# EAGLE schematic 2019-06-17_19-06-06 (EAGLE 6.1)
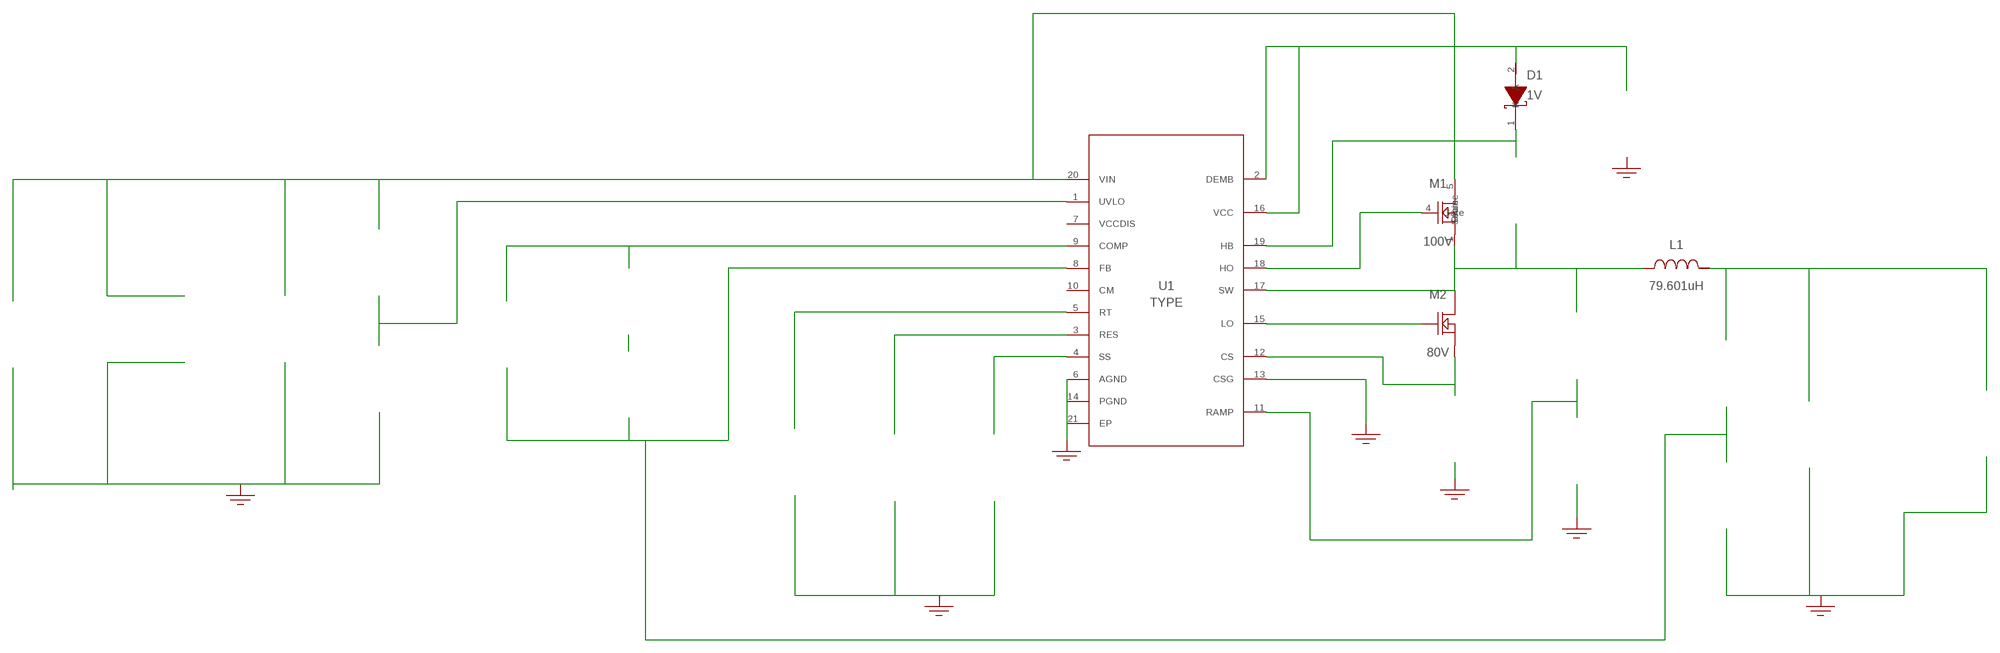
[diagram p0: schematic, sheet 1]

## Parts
CBOOT  100nF  GRM155R71A104KA01DGRM155R71A104KA01D  [0402]  (not placed on a sheet)
CCOMP1  820pF  CL05C821JB5NNNCCL05C821JB5NNNC  [0402]  (not placed on a sheet)
CCOMP2  680pF  GRM033R71C681KA01DGRM033R71C681KA01D  [0201]  (not placed on a sheet)
CIN  15uF  100SXV15M100SXV15M  [CAPSMT_62_E12]  (not placed on a sheet)
CIN_2  15uF  100SXV15M100SXV15M  [CAPSMT_62_E12]  (not placed on a sheet)
CINX  100nF  C2012X7R2A104K125AAC2012X7R2A104K125AA  [0805]  (not placed on a sheet)
COUT  22uF  EEE-FK1J220XPEEE-FK1J220XP  [SM_RADIAL_D8]  (not placed on a sheet)
CRAMP  820pF  GRM033R71E821KA01DGRM033R71E821KA01D  [0201]  (not placed on a sheet)
CRES  470nF  TMK212BJ474KD-TTMK212BJ474KD-T  [0805]  (not placed on a sheet)
CSS  15nF  CGA4F2C0G1H153J085AACGA4F2C0G1H153J085AA  [0805]  (not placed on a sheet)
CVCC  470nF  TMK212BJ474KD-TTMK212BJ474KD-T  [0805]  (not placed on a sheet)
D1  1V  CDBW46-GCDBW46-G  [SOD-123]
GND1  WB_GND  WB_GNDWB_GND  [WB_GND]
GND2  WB_GND  WB_GNDWB_GND  [WB_GND]
GND3  WB_GND  WB_GNDWB_GND  [WB_GND]
GND4  WB_GND  WB_GNDWB_GND  [WB_GND]
GND5  WB_GND  WB_GNDWB_GND  [WB_GND]
GND6  WB_GND  WB_GNDWB_GND  [WB_GND]
GND7  WB_GND  WB_GNDWB_GND  [WB_GND]
GND8  WB_GND  WB_GNDWB_GND  [WB_GND]
IOUT  WB_CURRENT_LOAD  WB_CURRENT_LOADWB_CURRENT_LOAD  [WB_CURRENT_LOAD]  (not placed on a sheet)
L1  79.601uH  CUSTOM1CUSTOM1  [GEN_Ind]
M1  100V  CSD19537Q3CSD19537Q3  [DQG0008A]
M2  80V  BSC117N08NS5ATMA1BSC117N08NS5ATMA1  [PG-TDSON-8]
RCOMP  40.2k  CRCW040240K2FKEDCRCW040240K2FKED  [0402]  (not placed on a sheet)
RFB1  910  RC0603FR-07910RLRC0603FR-07910RL  [0603]  (not placed on a sheet)
RFB2  47k  RC0603FR-0747KLRC0603FR-0747KL  [0603]  (not placed on a sheet)
RRAMP  806k  CRCW0603806KFKEACRCW0603806KFKEA  [0603]  (not placed on a sheet)
RSENSE  12m  CSR1206FK12L0CSR1206FK12L0  [1206]  (not placed on a sheet)
RT  9.31k  CRCW04029K31FKEDCRCW04029K31FKED  [0402]  (not placed on a sheet)
RUV1  1.3k  CRCW04021K30FKEDCRCW04021K30FKED  [0402]  (not placed on a sheet)
RUV2  54.9k  CRCW060354K9FKEACRCW060354K9FKEA  [0603]  (not placed on a sheet)
U1  LM5117PMHX/NOPB  LM5117PMHX/NOPBLM5117PMHX/NOPB  [PWP0020A]
VIN  WB_BATTERY  WB_BATTERYWB_BATTERY  [WB_BATTERY]  (not placed on a sheet)

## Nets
0: Cin.-@2 Cin_2.-@2 Cinx.2@2 Cout.-@2 Cramp.2@2 Cres.2@2 Css.2@2 Cvcc.2@2 GND1.1 GND2.1 GND3.1 GND4.1 GND5.1 GND6.1 GND7.1 GND8.1 Iout.-@2 Rfb1.2@2 Rsense.2@2 Rt.2@2 Ruv1.2@2 U1.6(AGND) U1.13(CSG) U1.14(PGND) U1.21(EP) Vin.-@2
1: Cvcc.1@1 D1.2(A) U1.2(DEMB) U1.16(VCC)
2: Ccomp2.2@2 Rcomp.2@2 Rfb1.1@1 Rfb2.2@2 U1.8(FB)
3: Cboot.2@2 L1.1 M1.1(Source) M1.2(Source) M1.3(Source) M2.5(Drain) M2.6(Drain) M2.7(Drain) M2.8(Drain) M2.9(Drain) Rramp.1@1 U1.17(SW)
4: Cboot.1@1 D1.1(K) U1.19(HB)
5: Cin.+@1 Cin_2.+@1 Cinx.1@1 M1.5(Drain) M1.6(Drain) M1.7(Drain) M1.8(Drain) M1.9(Drain) Ruv2.1@1 U1.20(VIN) Vin.+@1
6: Cramp.1@1 Rramp.2@2 U1.11(RAMP)
7: M2.1(Source) M2.2(Source) M2.3(Source) Rsense.1@1 U1.12(CS)
8: Cout.+@1 Iout.+@1 L1.2 Rfb2.1@1
9: Rt.1@1 U1.5(RT)
10: Ruv1.1@1 Ruv2.2@2 U1.1(UVLO)
11: Ccomp1.1@1 Ccomp2.1@1 U1.9(COMP)
12: Cres.1@1 U1.3(RES)
13: Css.1@1 U1.4(SS)
14: M1.4(Gate) U1.18(HO)
15: Ccomp1.2@2 Rcomp.1@1
16: M2.4(Gate) U1.15(LO)
Unconnected: CBOOT.1 CBOOT.2 CCOMP1.1 CCOMP1.2 CCOMP2.1 CCOMP2.2 CIN.1(+) CIN.2(-) CIN_2.1(+) CIN_2.2(-) CINX.1 CINX.2 COUT.1(+) COUT.2(-) CRAMP.1 CRAMP.2 CRES.1 CRES.2 CSS.1 CSS.2 CVCC.1 CVCC.2 IOUT.1(+) IOUT.2(-) RCOMP.1 RCOMP.2 RFB1.1 RFB1.2 RFB2.1 RFB2.2 RRAMP.1 RRAMP.2 RSENSE.1 RSENSE.2 RT.1 RT.2 RUV1.1 RUV1.2 RUV2.1 RUV2.2 U1.7(VCCDIS) U1.10(CM) VIN.1(+) VIN.2(-)

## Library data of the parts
CBOOT = AcceleratedDesigns_Lib:GRM155R71A104KA01D; Cap: 1.0E-7; ESR: 0.0; IRMS: 0.0; Manufacturer_Name: MuRata; Manufacturer_Part_Number: GRM155R71A104KA01D; VDC: 10.0; Vendor: MuRata
CCOMP1 = AcceleratedDesigns_Lib:CL05C821JB5NNNC; Cap: 8.2E-10; Datasheet_URL: http://www.samsungsem.com/servlet/FileDownload?type%3Dspec%26file%3DCL05C821JB5NNNC.pdf; ESR: 0.0; IRMS: 0.0; Manufacturer_Name: Samsung Electro-Mechanics; Manufacturer_Part_Number: CL05C821JB5NNNC; VDC: 50.0; Vendor: Samsung Electro-Mechanics
CCOMP2 = AcceleratedDesigns_Lib:GRM033R71C681KA01D; Cap: 6.8E-10; ESR: 0.0; IRMS: 0.0; Manufacturer_Name: MuRata; Manufacturer_Part_Number: GRM033R71C681KA01D; VDC: 16.0; Vendor: MuRata
CIN CIN_2 = AcceleratedDesigns_Lib:100SXV15M; Cap: 1.5E-5; Datasheet_URL: %20; ESR: 0.04; IRMS: 2.35; Manufacturer_Name: Panasonic; Manufacturer_Part_Number: 100SXV15M; VDC: 100.0; Vendor: Panasonic
CINX = AcceleratedDesigns_Lib:C2012X7R2A104K125AA; Cap: 1.0E-7; Datasheet_URL: https://product.tdk.com/en/search/capacitor/ceramic/mlcc/info?part%5Fno%3DC2012X7R2A104K125AA; ESR: 0.020726; IRMS: 1.456; Manufacturer_Name: TDK; Manufacturer_Part_Number: C2012X7R2A104K125AA; VDC: 100.0; Vendor: TDK
COUT = AcceleratedDesigns_Lib:EEE-FK1J220XP; Cap: 2.2E-5; Datasheet_URL: http://www.panasonic.com/industrial/components/pdf/smt%5Faec%5F050505.pdf; ESR: 1.2; IRMS: 0.12; Manufacturer_Name: Panasonic; Manufacturer_Part_Number: EEE-FK1J220XP; VDC: 63.0; Vendor: Panasonic
CRAMP = AcceleratedDesigns_Lib:GRM033R71E821KA01D; Cap: 8.2E-10; ESR: 0.0; IRMS: 0.0; Manufacturer_Name: MuRata; Manufacturer_Part_Number: GRM033R71E821KA01D; VDC: 25.0; Vendor: MuRata
CRES CVCC = AcceleratedDesigns_Lib:TMK212BJ474KD-T; Cap: 4.7E-7; ESR: 0.0; IRMS: 0.0; Manufacturer_Name: Taiyo Yuden; Manufacturer_Part_Number: TMK212BJ474KD-T; VDC: 20.0; Vendor: Taiyo Yuden
CSS = AcceleratedDesigns_Lib:CGA4F2C0G1H153J085AA; Cap: 1.5E-8; Datasheet_URL: http://product.tdk.com/capacitor/mlcc/en/documents/mlcc%5Fautomotive%5Fgeneral%5Fen.pdf; ESR: 0.0; IRMS: 0.0; Manufacturer_Name: TDK; Manufacturer_Part_Number: CGA4F2C0G1H153J085AA; VDC: 50.0; Vendor: TDK
D1 = AcceleratedDesigns_Lib:CDBW46-G; Datasheet_URL: http://www.comchiptech.com/cms/UserFiles/CDBW46%2DG%2520RevC.pdf; Io: 0.15; Manufacturer_Name: Comchip Technology; Manufacturer_Part_Number: CDBW46-G; VFatIo: 1.0; VRRM: 100.0; Vendor: Comchip Technology
GND1-GND8 = AcceleratedDesigns_Lib:WB_GND; Manufacturer_Name: WB_GND; Manufacturer_Part_Number: WB_GND; PowerPortType: POWER_GROUND; Value: Value
IOUT = AcceleratedDesigns_Lib:WB_CURRENT_LOAD; Manufacturer_Name: WB_CURRENT_LOAD; Manufacturer_Part_Number: WB_CURRENT_LOAD; PowerPortType: POWER_GROUND; Value: Value
L1 = AcceleratedDesigns_Lib:CUSTOM1; Component_Type: Inductor; Component_Type_Index: 20; DCR: 0.03; Dimension_X: 0.0; Dimension_Y: 0.0; Footprint: 0.00; Height: 0.0; IDC: 10.225; IDC_Max: 0.0; L: 7.960138860424252E-5; Manufacture: CUSTOM; Manufacturer_Name: CUSTOM; Manufacturer_Part_Number: GENERIC_INDUCTOR; Mount: ?; Part_ID: 18; Part_Number: CUSTOM; Price: 0.0; Quantity: 1; Quantity_In_stock: 0; Schematic_mapping_symbol: WB_INDUCTOR; Technology: ?; Thermal_ID: CUSTOM; Thermal_Status: N; Tolerance: 0.0; Vendor: Unknown
M1 = AcceleratedDesigns_Lib:CSD19537Q3; Datasheet_URL: http://www.ti.com/lit/ds/symlink/csd19537q3.pdf; IdsMax: 50.0; Manufacturer_Name: Texas Instruments; Manufacturer_Part_Number: CSD19537Q3; QgTyp: 16.0; Quantity: 1; Rdson45: 0.025; VdsMax: 100.0; Vendor: Texas Instruments
M2 = AcceleratedDesigns_Lib:BSC117N08NS5ATMA1; Datasheet_URL: http://www.infineon.com/dgdl/BSC123N08NS3G%5Frev2.3.pdf?folderId%3Ddb3a304313b8b5a60113cee8763b02d7%26fileId%3Ddb3a30431add1d95011ae80eb8555625; IdsMax: 55.0; Manufacturer_Name: Infineon Technologies; Manufacturer_Part_Number: BSC117N08NS5ATMA1; QgTyp: 19.0; Quantity: 1; Rdson45: 101.0; VdsMax: 80.0; Vendor: Infineon Technologies
RCOMP = AcceleratedDesigns_Lib:CRCW040240K2FKED; Manufacturer_Name: Vishay-Dale; Manufacturer_Part_Number: CRCW040240K2FKED; Power: 0.063; Resistance: 40200.0; Tolerance: 1.0; Vendor: Vishay-Dale
RFB1 = AcceleratedDesigns_Lib:RC0603FR-07910RL; Manufacturer_Name: Yageo; Manufacturer_Part_Number: RC0603FR-07910RL; Power: 0.1; Resistance: 910.0; Tolerance: 1.0; Vendor: Yageo America
RFB2 = AcceleratedDesigns_Lib:RC0603FR-0747KL; Manufacturer_Name: Yageo; Manufacturer_Part_Number: RC0603FR-0747KL; Power: 0.1; Resistance: 47000.0; Tolerance: 1.0; Vendor: Yageo America
RRAMP = AcceleratedDesigns_Lib:CRCW0603806KFKEA; Manufacturer_Name: Vishay-Dale; Manufacturer_Part_Number: CRCW0603806KFKEA; Power: 0.1; Resistance: 806000.0; Tolerance: 1.0; Vendor: Vishay-Dale
RSENSE = AcceleratedDesigns_Lib:CSR1206FK12L0; Manufacturer_Name: Stackpole Electronics Inc; Manufacturer_Part_Number: CSR1206FK12L0; Power: 0.5; Resistance: 0.012; Tolerance: 1.0; Vendor: Stackpole Electronics Inc
RT = AcceleratedDesigns_Lib:CRCW04029K31FKED; Manufacturer_Name: Vishay-Dale; Manufacturer_Part_Number: CRCW04029K31FKED; Power: 0.063; Resistance: 9310.0; Tolerance: 1.0; Vendor: Vishay-Dale
RUV1 = AcceleratedDesigns_Lib:CRCW04021K30FKED; Manufacturer_Name: Vishay-Dale; Manufacturer_Part_Number: CRCW04021K30FKED; Power: 0.063; Resistance: 1300.0; Tolerance: 1.0; Vendor: Vishay-Dale
RUV2 = AcceleratedDesigns_Lib:CRCW060354K9FKEA; Manufacturer_Name: Vishay-Dale; Manufacturer_Part_Number: CRCW060354K9FKEA; Power: 0.1; Resistance: 54900.0; Tolerance: 1.0; Vendor: Vishay-Dale
U1 = AcceleratedDesigns_Lib:LM5117PMHX/NOPB; Manufacturer: Texas Instruments; Manufacturer_Name: Texas Instruments; Manufacturer_Part_Number: LM5117PMHX/NOPB; PartNumber: LM5117PMHX/NOPB; RefDes: RefDes; TYPE: TYPE; Value: Value
VIN = AcceleratedDesigns_Lib:WB_BATTERY; Manufacturer_Name: WB_BATTERY; Manufacturer_Part_Number: WB_BATTERY; PowerPortType: POWER_GROUND; Value: Value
